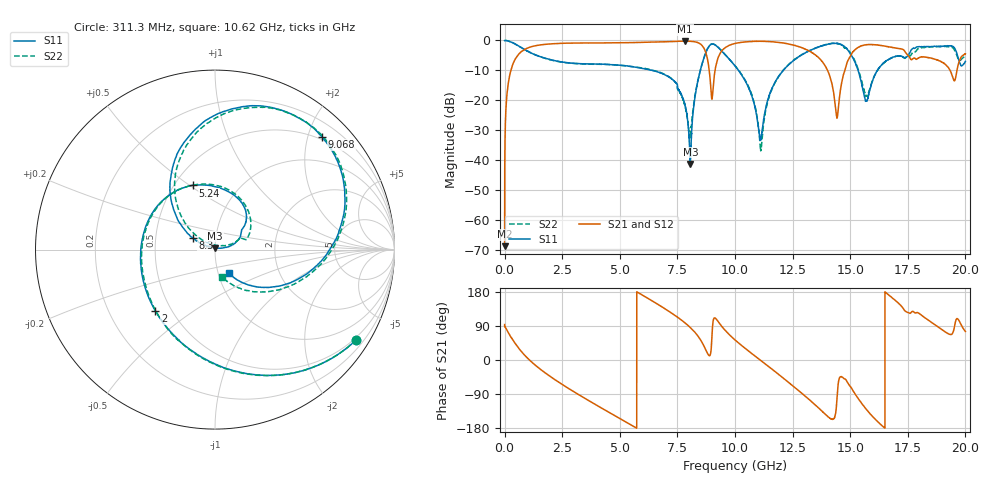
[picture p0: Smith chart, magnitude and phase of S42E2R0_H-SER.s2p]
!{S42E2R0}
!Johanson Technology Inc.
!www.johansontechnology.com
!Test Board Conditions:
!Substrate Type  RO4350B
!Substrate Thickness  50 mil
!Substrate Dk  3.66
!TL Type: GCPW
!TL Trace Width  60 mil
!TL Gap  10 mil
!Electrode orientation  Horizontal
!DUT TOPOLOGY	SERIES
!Mounting Pad LxW  14x55 mil
! Created Wed Nov 25 21:38:10 2020
# khz S ma R 50
! 2 Port Network Data from SP1.SP block
! freq  magS11  angS11  magS21  angS21  magS12  angS12  magS22  angS22
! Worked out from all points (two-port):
!   20001 points, 300 kHz to 20 GHz, reference 50 ohm
!   highest |S21| = -0.23 dB at 7.829 GHz (marker M1); lowest = -68.7 dB at 300 kHz (marker M2)
!   |S21| within 3 dB of the highest: 819.1 MHz to 8.692 GHz (7.873 GHz wide, 166 % of centre); 9.455 GHz to 13.15 GHz (3.693 GHz wide, 32.7 % of centre)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
!   lowest |S11| = -41.2 dB at 8.063 GHz (marker M3), VSWR 1.02, Z = 50 + j0.871 ohm
!   |S11| at or under -10 dB: 6.415 GHz to 8.496 GHz (2.08 GHz wide, 27.9 % of centre); 10.15 GHz to 12.09 GHz (1.941 GHz wide, 17.5 % of centre); 15.34 GHz to 16.18 GHz (837.5 MHz wide, 5.31 % of centre)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
!   |S22| runs from -36.9 to 0.0 dB; largest |S21 - S12| = 0.018
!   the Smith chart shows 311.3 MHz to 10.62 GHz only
!   S11 on the Smith chart (normalised r, x): 311.3 MHz: 0.43, -3.38; 2 GHz: 0.41, -0.36; 5.24 GHz: 0.62, +0.51; 8.3 GHz: 0.77, +0.10; 9.068 GHz: 0.44, +2.26; 10.62 GHz: 1.13, -0.30
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300  0.9954 -0.4  0.0003683 93.5  0.0004165 92.2  1 -0.3
112300  0.9894 -12.1  0.1374 77.6  0.1379 77.6  0.9898 -12.1
311300  0.9334 -32.5  0.3565 57.5  0.3576 57.5  0.9334 -32.5
2000300  0.4763 -134.1  0.8756 -44.3  0.8768 -44.3  0.4741 -134.4
3334300  0.4091 170.9  0.9074 -95.7  0.9074 -95.7  0.4063 177.6
5240300  0.3784 109.2  0.9183 -162.5  0.9181 -162.6  0.3772 106.5
6667300  0.2964 58.9  0.9456 146.3  0.9432 146.2  0.3003 55.9
7829300  0.08407 12.7  0.9737 97.9  0.9716 98.1  0.08117 19.4
8063300  0.008712 91.4  0.968 85.5  0.9668 85.7  0.02676 96.6
8300300  0.1405 152.8  0.9419 70.2  0.9426 70.3  0.1448 142.8
9068300  0.8672 46.5  0.1957 107.5  0.196 108.0  0.8705 45.1
1.00003e7  0.3767 -33.8  0.8896 53.0  0.8912 53.2  0.3783 -38.3
1.06213e7  0.152 -59.2  0.9569 22.1  0.9584 22.1  0.1587 -74.8
1.11293e7  0.02365 17.8  0.9688 -1.8  0.9672 -1.7  0.01494 168.0
1.17713e7  0.2122 54.6  0.9401 -32.2  0.9406 -32.1  0.2086 57.5
1.33343e7  0.7021 -19.4  0.628 -110.5  0.6343 -110.5  0.7034 -24.5
1.44253e7  0.8895 -93.9  0.0512 -102.8  0.05174 -103.1  0.8946 -93.6
1.56953e7  0.09901 -122.0  0.846 -129.5  0.8554 -129.5  0.1175 -126.9
1.66673e7  0.4824 -98.0  0.7853 172.1  0.7723 172.0  0.4798 -107.6
1.85813e7  0.7922 -172.3  0.4984 97.0  0.4986 97.5  0.7839 -174.2
1.95193e7  0.756 133.6  0.212 85.8  0.215 85.5  0.6983 132.2
2e7  0.4477 158.1  0.6009 75.1  0.6021 76.0  0.5449 139.6
